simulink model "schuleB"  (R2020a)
settings: Solver=FixedStepDiscrete  StartTime=0.0  StopTime=10.0  FixedStep=1  RelTol=1e-3  EnableMultiTasking=on

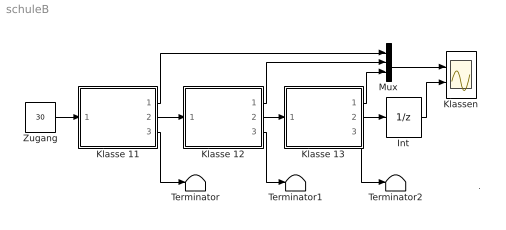
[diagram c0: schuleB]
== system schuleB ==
  note: .
  Int : UnitDelay  SampleTime=-1  HasFrameUpgradeWarning=on
  Klasse 11 : Subsystem  mask{x0=0, W=0.08, A=0.03}
      mask prompts: x0 "Anfangsstaerke"; W "Wiederholerrate"; A "Abbrecherrate"
  Klasse 12 : Subsystem  mask{x0=0, W=0.08, A=0.07}
      mask prompts: x0 "Anfangsstaerke"; W "Wiederholerrate"; A "Abbrecherrate"
  Klasse 13 : Subsystem  mask{x0=0, W=0.04, A=0.04}
      mask prompts: x0 "Anfangsstaerke"; W "Wiederholerrate"; A "Abbrecherrate"
  Klassen : Scope  NumInputPorts=2
  Mux : Mux  Inputs=3
  Terminator : Terminator
  Terminator1 : Terminator
  Terminator2 : Terminator
  Zugang : Constant  Value=30
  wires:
  Zugang/1 -> Klasse 11/1(neu)
  Klasse 11/2(versetzt) -> Klasse 12/1(neu)
  Klasse 12/2(versetzt) -> Klasse 13/1(neu)
  Klasse 13/2(versetzt) -> Int/1
  Mux/1 -> Klassen/1
  Klasse 11/1(Klassenstaerke) -> Mux/1
  Klasse 12/1(Klassenstaerke) -> Mux/2
  Klasse 13/1(Klassenstaerke) -> Mux/3
  Int/1 -> Klassen/2
  Klasse 11/3(abgegangen) -> Terminator/1
  Klasse 12/3(abgegangen) -> Terminator1/1
  Klasse 13/3(abgegangen) -> Terminator2/1

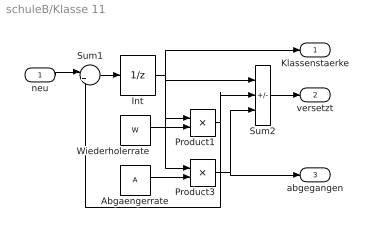
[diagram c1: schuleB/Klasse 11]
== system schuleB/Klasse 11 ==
  note: .
  neu : Inport
  Abgaengerrate : Constant  Value=A
  Int : UnitDelay  InitialCondition=x0  SampleTime=-1  HasFrameUpgradeWarning=on
  Product1 : Product  InputSameDT=on  RndMeth=Zero  SaturateOnIntegerOverflow=on
  Product3 : Product  InputSameDT=on  RndMeth=Zero  SaturateOnIntegerOverflow=on
  Sum1 : Sum  Inputs=|++  InputSameDT=on  SaturateOnIntegerOverflow=on
  Sum2 : Sum  Inputs=+--  InputSameDT=on  SaturateOnIntegerOverflow=on
  Wiederholerrate : Constant  Value=W
  Klassenstaerke : Outport
  versetzt : Outport  Port=2
  abgegangen : Outport  Port=3
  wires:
  Sum2/1 -> versetzt/1
  neu/1 -> Sum1/1
  Product3/1 -> Sum2/3, abgegangen/1
  Product1/1 -> Sum2/2, Sum1/2
  Abgaengerrate/1 -> Product3/2
  Int/1 -> Sum2/1, Product3/1, Product1/1, Klassenstaerke/1
  Wiederholerrate/1 -> Product1/2
  Sum1/1 -> Int/1

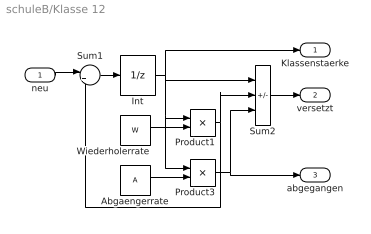
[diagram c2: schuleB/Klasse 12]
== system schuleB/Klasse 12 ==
  neu : Inport
  Abgaengerrate : Constant  Value=A
  Int : UnitDelay  InitialCondition=x0  SampleTime=-1  HasFrameUpgradeWarning=on
  Product1 : Product  InputSameDT=on  RndMeth=Zero  SaturateOnIntegerOverflow=on
  Product3 : Product  InputSameDT=on  RndMeth=Zero  SaturateOnIntegerOverflow=on
  Sum1 : Sum  Inputs=|++  InputSameDT=on  SaturateOnIntegerOverflow=on
  Sum2 : Sum  Inputs=+--  InputSameDT=on  SaturateOnIntegerOverflow=on
  Wiederholerrate : Constant  Value=W
  Klassenstaerke : Outport
  versetzt : Outport  Port=2
  abgegangen : Outport  Port=3
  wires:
  Sum1/1 -> Int/1
  Wiederholerrate/1 -> Product1/2
  Int/1 -> Klassenstaerke/1, Product1/1, Product3/1, Sum2/1
  Abgaengerrate/1 -> Product3/2
  Product1/1 -> Sum1/2, Sum2/2
  Product3/1 -> abgegangen/1, Sum2/3
  neu/1 -> Sum1/1
  Sum2/1 -> versetzt/1

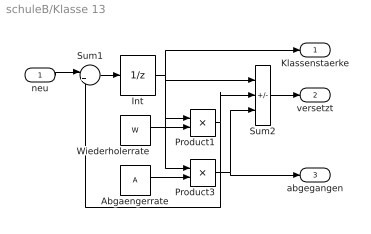
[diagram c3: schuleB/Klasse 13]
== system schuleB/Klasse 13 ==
  neu : Inport
  Abgaengerrate : Constant  Value=A
  Int : UnitDelay  InitialCondition=x0  SampleTime=-1  HasFrameUpgradeWarning=on
  Product1 : Product  InputSameDT=on  RndMeth=Zero  SaturateOnIntegerOverflow=on
  Product3 : Product  InputSameDT=on  RndMeth=Zero  SaturateOnIntegerOverflow=on
  Sum1 : Sum  Inputs=|++  InputSameDT=on  SaturateOnIntegerOverflow=on
  Sum2 : Sum  Inputs=+--  InputSameDT=on  SaturateOnIntegerOverflow=on
  Wiederholerrate : Constant  Value=W
  Klassenstaerke : Outport
  versetzt : Outport  Port=2
  abgegangen : Outport  Port=3
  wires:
  Sum2/1 -> versetzt/1
  neu/1 -> Sum1/1
  Product3/1 -> Sum2/3, abgegangen/1
  Product1/1 -> Sum2/2, Sum1/2
  Abgaengerrate/1 -> Product3/2
  Int/1 -> Sum2/1, Product3/1, Product1/1, Klassenstaerke/1
  Wiederholerrate/1 -> Product1/2
  Sum1/1 -> Int/1
